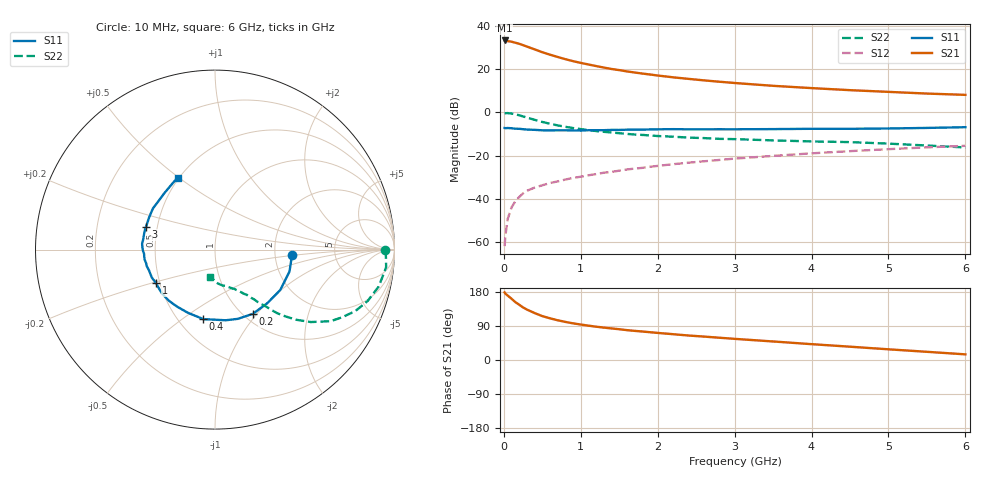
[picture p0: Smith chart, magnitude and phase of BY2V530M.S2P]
! SIEMENS Small Signal Semiconductors
! BFY420
! Si NPN RF SIEGET Grounded Emitter Transistor in MICRO-X
! VCE = 2.5 V  IC = 30 mA
! Common Emitter S-Parameters:  October  1996
# GHz  S  MA  R  50
!  f  S11  S21  S12  S22
! GHz  MAG  ANG  MAG  ANG  MAG  ANG  MAG  ANG
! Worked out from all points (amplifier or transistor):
!   36 points, 10 MHz to 6 GHz, reference 50 ohm
!   highest |S21| = 33.2 dB at 10 MHz (marker M1)
!   |S21| within 3 dB of that: start of sweep to 313.4 MHz
!   unconditionally stable (mu >= 1): 1.659 GHz to end of sweep
!   at 250 MHz: K = 0.36, MSG = 34.3 dB, |S12| = -37.5 dB
!   at 1.4 GHz: K = 0.97, MSG = 23.8 dB, |S12| = -27.6 dB
!   at 6 GHz: K = 1.07, MAG = 10.2 dB, |S12| = -15.5 dB
!   S11 on the Smith chart (normalised r, x): 10 MHz: 2.51, -0.17; 200 MHz: 1.10, -0.95; 400 MHz: 0.66, -0.60; 1 GHz: 0.48, -0.21; 3 GHz: 0.43, +0.13; 6 GHz: 0.49, +0.49
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0.01  0.4322 -3.7  45.89 178.3  0.0008 136.9  0.9494 -0.2
0.02  0.4292 -6.6  45.48 175.2  0.0014 93.9  0.9523 -1.6
0.1  0.4278 -31.7  42.98 161.7  0.0063 80.9  0.9352 -12.7
0.15  0.4172 -45.7  40.63 152.6  0.0088 73.7  0.8975 -18.6
0.2  0.4155 -59.4  38.44 145.8  0.011 71.2  0.8533 -23.7
0.25  0.4063 -71.7  35.71 138.7  0.0133 68.4  0.8016 -28.1
0.3  0.3982 -81.4  33.15 133.0  0.0153 66.2  0.7571 -31.8
0.4  0.3927 -99.6  28.56 123.9  0.0181 63.8  0.6692 -37.1
0.5  0.383 -113.2  24.53 115.8  0.0205 62.0  0.5983 -40.8
0.6  0.3815 -123.3  21.5 110.0  0.0231 61.1  0.5424 -43.4
0.7  0.3836 -131.9  19.04 104.8  0.0252 61.7  0.4985 -45.5
0.8  0.3838 -139.6  16.92 100.5  0.0278 60.8  0.4615 -46.9
1  0.3779 -150.5  13.88 93.6  0.0323 61.7  0.4087 -49.0
1.1  0.3848 -156.0  12.76 90.6  0.0349 62.5  0.3872 -50.3
1.3  0.3856 -162.7  10.83 85.5  0.04 62.1  0.3535 -51.8
1.6  0.3959 -171.8  8.827 78.8  0.0475 62.0  0.3162 -54.4
2.2  0.4074 175.5  6.443 68.1  0.063 59.7  0.2726 -59.4
3  0.4046 161.9  4.762 55.8  0.0848 55.2  0.2394 -65.4
3.5  0.4085 153.9  4.096 48.9  0.0981 51.5  0.2238 -69.5
4.5  0.4148 139.5  3.25 35.1  0.1263 43.4  0.2042 -78.2
5.5  0.4351 124.1  2.711 21.6  0.1545 33.9  0.1704 -91.7
6  0.4521 117.5  2.53 14.9  0.1676 29.0  0.1537 -101.1
